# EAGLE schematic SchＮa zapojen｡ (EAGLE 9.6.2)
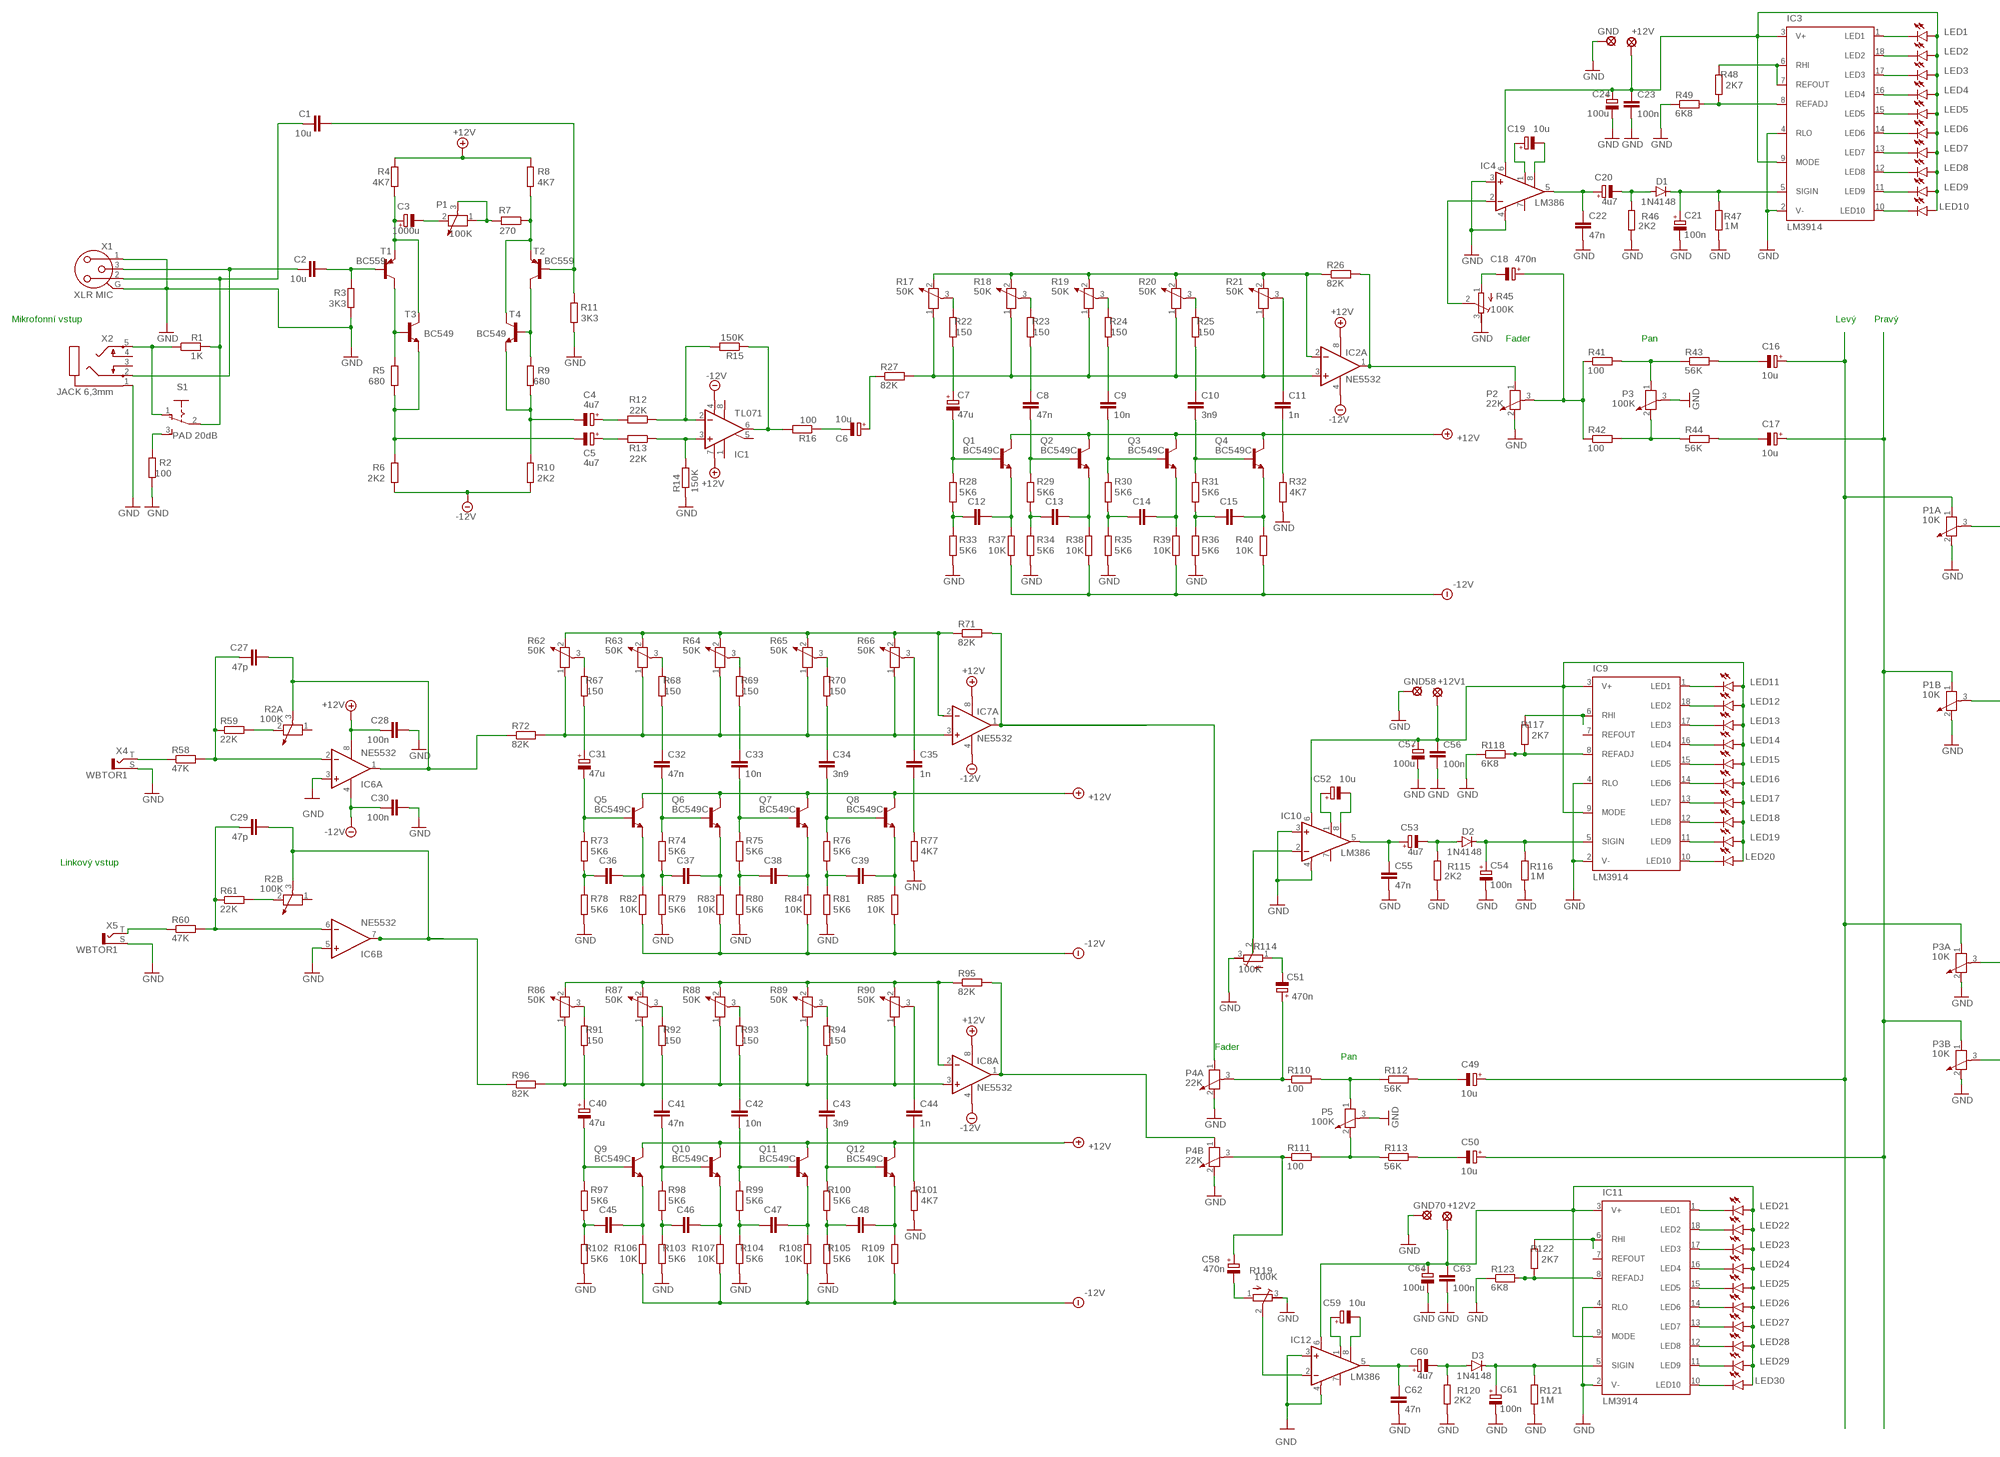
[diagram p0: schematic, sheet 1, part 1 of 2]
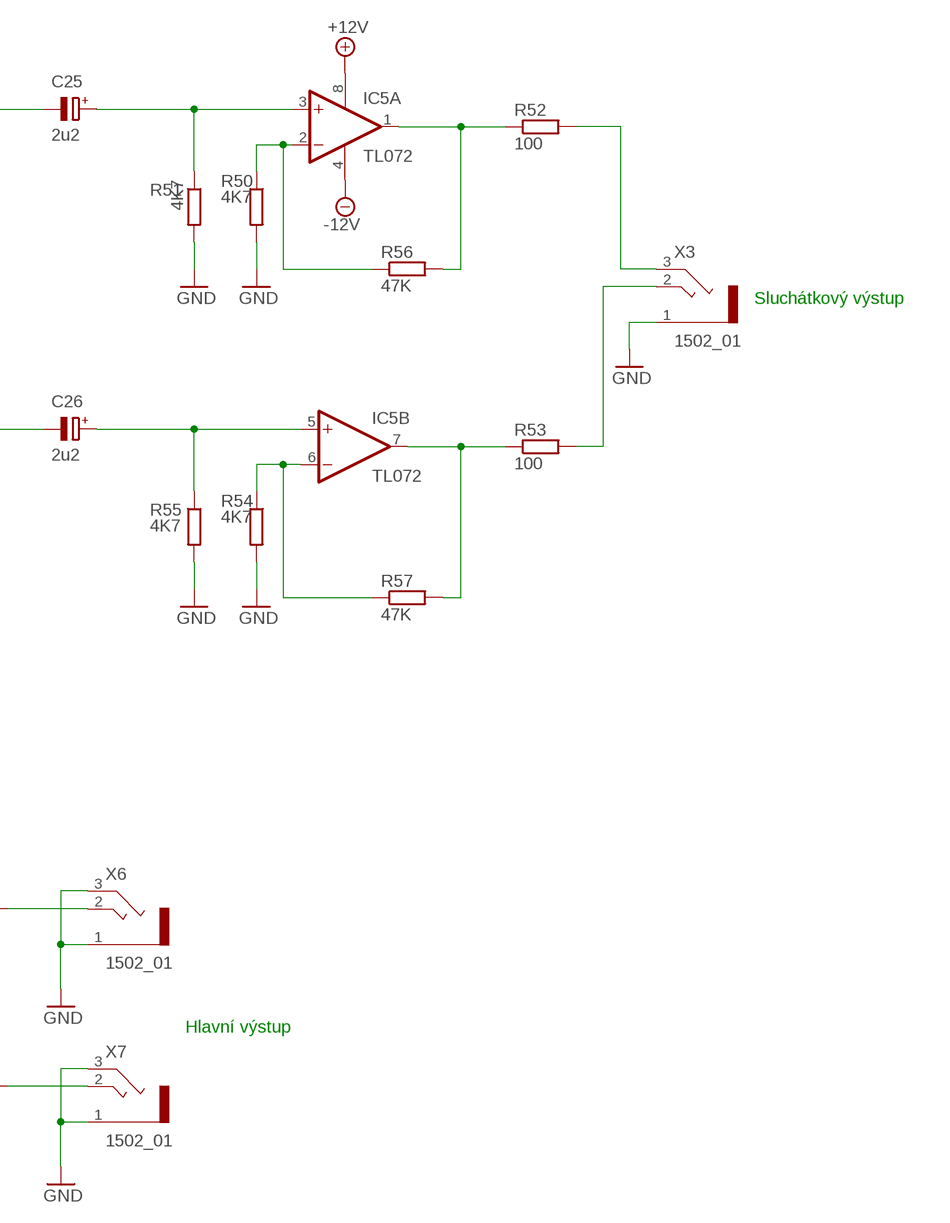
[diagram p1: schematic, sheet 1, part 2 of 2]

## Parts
+12V  MCS08  [MCS08]
+12V1  MCS08  [MCS08]
+12V2  MCS08  [MCS08]
C1  10u  C-EU050-025X075  [C050-025X075]
C2  10u  C-EU050-025X075  [C050-025X075]
C3  1000u  CPOL-EUE3.5-8  [E3,5-8]
C4  4u7  CPOL-EUE3.5-8  [E3,5-8]
C5  4u7  CPOL-EUE3.5-8  [E3,5-8]
C6  10u  CPOL-EUE3.5-8  [E3,5-8]
C7  47u  CPOL-EUE1.8-4  [E1,8-4]
C8  47n  C-EU050-030X075  [C050-030X075]
C9  10n  C-EU050-030X075  [C050-030X075]
C10  3n9  C-EU050-030X075  [C050-030X075]
C11  1n  C-EU050-030X075  [C050-030X075]
C12  C-EU050-030X075  [C050-030X075]
C13  C-EU050-030X075  [C050-030X075]
C14  C-EU050-030X075  [C050-030X075]
C15  C-EU050-030X075  [C050-030X075]
C16  10u  CPOL-EUE2.5-5  [E2,5-5]
C17  10u  CPOL-EUE2.5-5  [E2,5-5]
C18  470n  CPOL-EUE2.5-5  [E2,5-5]
C19  10u  CPOL-EUE2.5-5  [E2,5-5]
C20  4u7  CPOL-EUE2.5-5  [E2,5-5]
C21  100n  CPOL-EUE2.5-5  [E2,5-5]
C22  47n  C-EU050-030X075  [C050-030X075]
C23  100n  C-EU050-030X075  [C050-030X075]
C24  100u  CPOL-EUE2.5-5  [E2,5-5]
C25  2u2  CPOL-EUE2,5-6E  [E2,5-6E]
C26  2u2  CPOL-EUE2,5-6E  [E2,5-6E]
C27  47p  C-EU050-024X044  [C050-024X044]
C28  100n  C-EU050-024X044  [C050-024X044]
C29  47p  C-EU050-024X044  [C050-024X044]
C30  100n  C-EU050-024X044  [C050-024X044]
C31  47u  CPOL-EUE1.8-4  [E1,8-4]
C32  47n  C-EU050-030X075  [C050-030X075]
C33  10n  C-EU050-030X075  [C050-030X075]
C34  3n9  C-EU050-030X075  [C050-030X075]
C35  1n  C-EU050-030X075  [C050-030X075]
C36  C-EU050-030X075  [C050-030X075]
C37  C-EU050-030X075  [C050-030X075]
C38  C-EU050-030X075  [C050-030X075]
C39  C-EU050-030X075  [C050-030X075]
C40  47u  CPOL-EUE1.8-4  [E1,8-4]
C41  47n  C-EU050-030X075  [C050-030X075]
C42  10n  C-EU050-030X075  [C050-030X075]
C43  3n9  C-EU050-030X075  [C050-030X075]
C44  1n  C-EU050-030X075  [C050-030X075]
C45  C-EU050-030X075  [C050-030X075]
C46  C-EU050-030X075  [C050-030X075]
C47  C-EU050-030X075  [C050-030X075]
C48  C-EU050-030X075  [C050-030X075]
C49  10u  CPOL-EUE2.5-5  [E2,5-5]
C50  10u  CPOL-EUE2.5-5  [E2,5-5]
C51  470n  CPOL-EUE2.5-5  [E2,5-5]
C52  10u  CPOL-EUE2.5-5  [E2,5-5]
C53  4u7  CPOL-EUE2.5-5  [E2,5-5]
C54  100n  CPOL-EUE2.5-5  [E2,5-5]
C55  47n  C-EU050-030X075  [C050-030X075]
C56  100n  C-EU050-030X075  [C050-030X075]
C57  100u  CPOL-EUE2.5-5  [E2,5-5]
C58  470n  CPOL-EUE2.5-5  [E2,5-5]
C59  10u  CPOL-EUE2.5-5  [E2,5-5]
C60  4u7  CPOL-EUE2.5-5  [E2,5-5]
C61  100n  CPOL-EUE2.5-5  [E2,5-5]
C62  47n  C-EU050-030X075  [C050-030X075]
C63  100n  C-EU050-030X075  [C050-030X075]
C64  100u  CPOL-EUE2.5-5  [E2,5-5]
D1  1N4148  1N4148DO35-7  [DO35-7]
D2  1N4148  1N4148DO35-7  [DO35-7]
D3  1N4148  1N4148DO35-7  [DO35-7]
GND  MCS08  [MCS08]
GND58  MCS08  [MCS08]
GND70  MCS08  [MCS08]
IC1  TL071  TL071P  [DIL08]
IC2  NE5532  NE5532N  [DIL08]
IC3  LM3914  LM3914N  [DIL18]
IC4  LM386  LM386N-1  [DIL08]
IC5  TL072  TL072P  [DIL08]
IC6  NE5532  NE5532N  [DIL08]
IC7  NE5532  NE5532N  [DIL08]
IC8  NE5532  NE5532N  [DIL08]
IC9  LM3914  LM3914N  [DIL18]
IC10  LM386  LM386N-1  [DIL08]
IC11  LM3914  LM3914N  [DIL18]
IC12  LM386  LM386N-1  [DIL08]
LED1  LED10MM  [LED10MM]
LED2  LED10MM  [LED10MM]
LED3  LED10MM  [LED10MM]
LED4  LED10MM  [LED10MM]
LED5  LED10MM  [LED10MM]
LED6  LED10MM  [LED10MM]
LED7  LED10MM  [LED10MM]
LED8  LED10MM  [LED10MM]
LED9  LED10MM  [LED10MM]
LED10  LED10MM  [LED10MM]
LED11  LED10MM  [LED10MM]
LED12  LED10MM  [LED10MM]
LED13  LED10MM  [LED10MM]
LED14  LED10MM  [LED10MM]
LED15  LED10MM  [LED10MM]
LED16  LED10MM  [LED10MM]
LED17  LED10MM  [LED10MM]
LED18  LED10MM  [LED10MM]
LED19  LED10MM  [LED10MM]
LED20  LED10MM  [LED10MM]
LED21  LED10MM  [LED10MM]
LED22  LED10MM  [LED10MM]
LED23  LED10MM  [LED10MM]
LED24  LED10MM  [LED10MM]
LED25  LED10MM  [LED10MM]
LED26  LED10MM  [LED10MM]
LED27  LED10MM  [LED10MM]
LED28  LED10MM  [LED10MM]
LED29  LED10MM  [LED10MM]
LED30  LED10MM  [LED10MM]
P1  100K  POTENTIOMETER_PT-10  [PT-10]
P1A  10K  POTENTIOMETER_PT-10  [PT-10]
P1B  10K  POTENTIOMETER_PT-10  [PT-10]
P2  22K  POTENTIOMETER_PT-10  [PT-10]
P3  100K  POTENTIOMETER_PT-10  [PT-10]
P3A  10K  POTENTIOMETER_PT-10  [PT-10]
P3B  10K  POTENTIOMETER_PT-10  [PT-10]
P4A  22K  POTENTIOMETER_PT-10  [PT-10]
P4B  22K  POTENTIOMETER_PT-10  [PT-10]
P5  100K  POTENTIOMETER_PT-10  [PT-10]
Q1  BC549C  [TO92-EBC]
Q2  BC549C  [TO92-EBC]
Q3  BC549C  [TO92-EBC]
Q4  BC549C  [TO92-EBC]
Q5  BC549C  [TO92-EBC]
Q6  BC549C  [TO92-EBC]
Q7  BC549C  [TO92-EBC]
Q8  BC549C  [TO92-EBC]
Q9  BC549C  [TO92-EBC]
Q10  BC549C  [TO92-EBC]
Q11  BC549C  [TO92-EBC]
Q12  BC549C  [TO92-EBC]
R1  1K  R-EU_0207/7  [0207/7]
R2  100  R-EU_0207/7  [0207/7]
R2A  100K  POTENTIOMETER_PT-10  [PT-10]
R2B  100K  POTENTIOMETER_PT-10  [PT-10]
R3  3K3  R-EU_0207/7  [0207/7]
R4  4K7  R-EU_0207/7  [0207/7]
R5  680  R-EU_0207/7  [0207/7]
R6  2K2  R-EU_0207/7  [0207/7]
R7  270  R-EU_0207/7  [0207/7]
R8  4K7  R-EU_0207/7  [0207/7]
R9  680  R-EU_0207/7  [0207/7]
R10  2K2  R-EU_0207/7  [0207/7]
R11  3K3  R-EU_0207/7  [0207/7]
R12  22K  R-EU_0207/7  [0207/7]
R13  22K  R-EU_0207/7  [0207/7]
R14  150K  R-EU_0207/7  [0207/7]
R15  150K  R-EU_0207/7  [0207/7]
R16  100  R-EU_0207/7  [0207/7]
R17  50K  POTENTIOMETER_PT-10S  [PT-10S]
R18  50K  POTENTIOMETER_PT-10S  [PT-10S]
R19  50K  POTENTIOMETER_PT-10S  [PT-10S]
R20  50K  POTENTIOMETER_PT-10S  [PT-10S]
R21  50K  POTENTIOMETER_PT-10S  [PT-10S]
R22  150  R-EU_0207/7  [0207/7]
R23  150  R-EU_0207/7  [0207/7]
R24  150  R-EU_0207/7  [0207/7]
R25  150  R-EU_0207/7  [0207/7]
R26  82K  R-EU_0207/7  [0207/7]
R27  82K  R-EU_0207/7  [0207/7]
R28  5K6  R-EU_0207/7  [0207/7]
R29  5K6  R-EU_0207/7  [0207/7]
R30  5K6  R-EU_0207/7  [0207/7]
R31  5K6  R-EU_0207/7  [0207/7]
R32  4K7  R-EU_0207/7  [0207/7]
R33  5K6  R-EU_0207/7  [0207/7]
R34  5K6  R-EU_0207/7  [0207/7]
R35  5K6  R-EU_0207/7  [0207/7]
R36  5K6  R-EU_0207/7  [0207/7]
R37  10K  R-EU_0207/7  [0207/7]
R38  10K  R-EU_0207/7  [0207/7]
R39  10K  R-EU_0207/7  [0207/7]
R40  10K  R-EU_0207/7  [0207/7]
R41  100  R-EU_0207/10  [0207/10]
R42  100  R-EU_0207/10  [0207/10]
R43  56K  R-EU_0207/10  [0207/10]
R44  56K  R-EU_0207/10  [0207/10]
R45  100K  R-TRIMM74W  [RTRIM74W]
R46  2K2  R-EU_0204/7  [0204/7]
R47  1M  R-EU_0204/7  [0204/7]
R48  2K7  R-EU_0204/7  [0204/7]
R49  6K8  R-EU_0204/7  [0204/7]
R50  4K7  R-EU_0207/7  [0207/7]
R51  4K7  R-EU_0207/7  [0207/7]
R52  100  R-EU_0207/7  [0207/7]
R53  100  R-EU_0207/7  [0207/7]
R54  4K7  R-EU_0207/7  [0207/7]
R55  4K7  R-EU_0207/7  [0207/7]
R56  47K  R-EU_0207/7  [0207/7]
R57  47K  R-EU_0207/7  [0207/7]
R58  47K  R-EU_0207/7  [0207/7]
R59  22K  R-EU_0207/7  [0207/7]
R60  47K  R-EU_0207/7  [0207/7]
R61  22K  R-EU_0207/7  [0207/7]
R62  50K  POTENTIOMETER_PT-10S  [PT-10S]
R63  50K  POTENTIOMETER_PT-10S  [PT-10S]
R64  50K  POTENTIOMETER_PT-10S  [PT-10S]
R65  50K  POTENTIOMETER_PT-10S  [PT-10S]
R66  50K  POTENTIOMETER_PT-10S  [PT-10S]
R67  150  R-EU_0207/7  [0207/7]
R68  150  R-EU_0207/7  [0207/7]
R69  150  R-EU_0207/7  [0207/7]
R70  150  R-EU_0207/7  [0207/7]
R71  82K  R-EU_0207/7  [0207/7]
R72  82K  R-EU_0207/7  [0207/7]
R73  5K6  R-EU_0207/7  [0207/7]
R74  5K6  R-EU_0207/7  [0207/7]
R75  5K6  R-EU_0207/7  [0207/7]
R76  5K6  R-EU_0207/7  [0207/7]
R77  4K7  R-EU_0207/7  [0207/7]
R78  5K6  R-EU_0207/7  [0207/7]
R79  5K6  R-EU_0207/7  [0207/7]
R80  5K6  R-EU_0207/7  [0207/7]
R81  5K6  R-EU_0207/7  [0207/7]
R82  10K  R-EU_0207/7  [0207/7]
R83  10K  R-EU_0207/7  [0207/7]
R84  10K  R-EU_0207/7  [0207/7]
R85  10K  R-EU_0207/7  [0207/7]
R86  50K  POTENTIOMETER_PT-10S  [PT-10S]
R87  50K  POTENTIOMETER_PT-10S  [PT-10S]
R88  50K  POTENTIOMETER_PT-10S  [PT-10S]
R89  50K  POTENTIOMETER_PT-10S  [PT-10S]
R90  50K  POTENTIOMETER_PT-10S  [PT-10S]
R91  150  R-EU_0207/7  [0207/7]
R92  150  R-EU_0207/7  [0207/7]
R93  150  R-EU_0207/7  [0207/7]
R94  150  R-EU_0207/7  [0207/7]
R95  82K  R-EU_0207/7  [0207/7]
R96  82K  R-EU_0207/7  [0207/7]
R97  5K6  R-EU_0207/7  [0207/7]
R98  5K6  R-EU_0207/7  [0207/7]
R99  5K6  R-EU_0207/7  [0207/7]
R100  5K6  R-EU_0207/7  [0207/7]
R101  4K7  R-EU_0207/7  [0207/7]
R102  5K6  R-EU_0207/7  [0207/7]
R103  5K6  R-EU_0207/7  [0207/7]
R104  5K6  R-EU_0207/7  [0207/7]
R105  5K6  R-EU_0207/7  [0207/7]
R106  10K  R-EU_0207/7  [0207/7]
R107  10K  R-EU_0207/7  [0207/7]
R108  10K  R-EU_0207/7  [0207/7]
R109  10K  R-EU_0207/7  [0207/7]
R110  100  R-EU_0207/10  [0207/10]
R111  100  R-EU_0207/10  [0207/10]
R112  56K  R-EU_0207/10  [0207/10]
R113  56K  R-EU_0207/10  [0207/10]
R114  100K  R-TRIMM74W  [RTRIM74W]
R115  2K2  R-EU_0204/7  [0204/7]
R116  1M  R-EU_0204/7  [0204/7]
R117  2K7  R-EU_0204/7  [0204/7]
R118  6K8  R-EU_0204/7  [0204/7]
R119  100K  R-TRIMM74W  [RTRIM74W]
R120  2K2  R-EU_0204/7  [0204/7]
R121  1M  R-EU_0204/7  [0204/7]
R122  2K7  R-EU_0204/7  [0204/7]
R123  6K8  R-EU_0204/7  [0204/7]
S1  PAD 20dB  255SB  [255SB]
T1  BC559  BC559A-PNP-TO92-EBC  [TO92-EBC]
T2  BC559  BC559A-PNP-TO92-EBC  [TO92-EBC]
T3  BC549  BC549-NPN-TO92-CBE  [TO92-CBE]
T4  BC549  BC549-NPN-TO92-CBE  [TO92-CBE]
X1  XLR MIC  NC3FAV2  [NC3FAV2]
X2  JACK 6,3mm  PG203J  [PG203J]
X3  1502_01  [1502_01]
X4  WBTOR1  [WBTOR1]
X5  WBTOR1  [WBTOR1]
X6  1502_01  [1502_01]
X7  1502_01  [1502_01]

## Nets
+12V: C28.1 IC1.7(V+) IC2.8(P:V+) IC5.8(P:V+) IC6.8(P:V+) IC7.8(P:V+) IC8.8(P:V+) R4.2 R8.2
-12V: C30.1 IC1.4(V-) IC2.4(P:V-) IC5.4(P:V-) IC6.4(P:V-) IC7.4(P:V-) IC8.4(P:V-) R6.1 R10.1
GND: C21.- C22.2 C23.2 C24.- C28.2 C30.2 C54.- C55.2 C61.- C62.2 GND.MP IC3.2(V-) IC3.4(RLO) IC4.3(+IN) IC4.4(GND) IC6.3(A:+IN) IC6.5(B:+IN) P1A.2 P1B.2 P2.2 P3.3 P3A.2 P3B.2 P4A.2 P4B.2 P5.3 R2.1 R3.1 R11.1 R14.1 R32.1 R33.1 R34.1 R35.1 R36.1 R45.3(E) R46.1 R47.1 R49.1 R50.2 R51.2 R54.2 R55.2 R77.1 R78.1 R79.1 R80.1 R81.1 R101.1 R102.1 R103.1 R104.1 R105.1 R114.3(E) R115.1 R116.1 R119.3(E) R120.1 R121.1 X1.1 X1.G X2.1 X3.1 X4.S X5.S X6.1 X6.3 X7.1 X7.3
GND1: C56.2 C57.- GND58.MP IC9.2(V-) IC9.4(RLO) IC10.3(+IN) IC10.4(GND) R118.1 ; supply symbol labelled GND
GND2: C63.2 C64.- GND70.MP IC11.2(V-) IC11.4(RLO) IC12.3(+IN) IC12.4(GND) R123.1 ; supply symbol labelled GND
N$1: C6.+ R27.1
N$2: R2.2 S1.3(S)
N$3: C2.1 X1.3 X2.2
N$4: C1.1 R1.2 S1.2(P) X1.2
N$5: R1.1 S1.1(O) X2.5
N$6: R17.3 R22.2
N$7: C2.2 R3.2 T1.B
N$8: R5.2 T1.C T3.B
N$9: R9.2 T2.C T4.B
N$10: C1.2 R11.2 T2.B
N$11: R18.3 R23.2
N$12: R7.1 R8.1 T2.E T4.C
N$13: C3.+ R4.1 T1.E T3.C
N$14: C5.- R5.1 R6.2 T3.E
N$15: R19.3 R24.2
N$16: C4.- R9.1 R10.2 T4.E
N$17: C3.- P1.2
N$18: P1.1 P1.3 R7.2
N$19: C4.+ R12.2
N$20: C5.+ R13.2
N$21: IC1.2(-IN) R12.1 R15.2
N$22: IC1.3(+IN) R13.1 R14.2
N$23: C6.- R16.1
N$24: IC1.6(OUT) R15.1 R16.2
N$25: R20.3 R25.2
N$26: C7.+ R22.1
N$27: R17.1 R18.1 R19.1 R20.1 R21.1 R27.2
N$28: C8.1 R23.1
N$29: C9.1 R24.1
N$30: C10.1 R25.1
N$31: C7.- Q1.B R28.2
N$32: C8.2 Q2.B R29.2
N$33: C9.2 Q3.B R30.2
N$34: C10.2 Q4.B R31.2
N$35: C15.2 Q4.E R40.2
N$36: C14.2 Q3.E R39.2
N$37: C13.2 Q2.E R38.2
N$38: C12.2 Q1.E R37.2
N$39: C12.1 R28.1 R33.2
N$40: C13.1 R29.1 R34.2
N$41: C14.1 R30.1 R35.2
N$42: C15.1 R31.1 R36.2
N$43: C11.2 R32.2
N$44: R17.2 R18.2 R19.2 R20.2 R21.2 R26.1
N$45: Q1.C Q2.C Q3.C Q4.C
N$46: R37.1 R38.1 R39.1 R40.1
N$47: C51.+ P4A.3 R110.1
N$48: IC2.1(A:OUT) P2.1 R26.2
N$49: C11.1 R21.3
N$50: P3A.3 X6.2
N$51: P3.1 R41.2 R43.1
N$52: P3.2 R42.2 R44.1
N$53: C16.- R43.2
N$54: C17.- R44.2
N$55: P3B.3 X7.2
N$56: R62.3 R67.2
N$57: C58.+ P4B.3 R111.1
N$58: C19.+ IC4.1(GAIN)
N$59: C19.- IC4.8(GAIN)
N$60: C20.+ C22.1 IC4.5(OUT)
N$61: C20.- D1.A R46.2
N$62: C21.+ D1.C IC3.5(SIGIN) R47.2
N$63: IC4.2(-IN) R45.2(S)
N$64: C18.- R45.1(A)
N$65: C18.+ P2.3 R41.1 R42.1
N$66: IC3.8(REFADJ) R48.1 R49.2
N$67: IC3.6(RHI) IC3.7(REFOUT) R48.2
N$68: +12V.MP C23.1 C24.+ IC3.3(V+) IC3.9(MODE) IC4.6(VS) LED1.A LED2.A LED3.A LED4.A LED5.A LED6.A LED7.A LED8.A LED9.A LED10.A
N$69: IC3.1(LED1) LED1.K(C)
N$70: IC3.18(LED2) LED2.K(C)
N$71: IC3.17(LED3) LED3.K(C)
N$72: IC3.16(LED4) LED4.K(C)
N$73: IC3.15(LED5) LED5.K(C)
N$74: IC3.14(LED6) LED6.K(C)
N$75: IC3.13(LED7) LED7.K(C)
N$76: IC3.12(LED8) LED8.K(C)
N$77: IC3.11(LED9) LED9.K(C)
N$78: IC3.10(LED10) LED10.K(C)
N$79: C26.- P1B.3
N$80: C25.- P1A.3
N$81: C25.+ IC5.3(A:+IN) R51.1
N$82: C26.+ IC5.5(B:+IN) R55.1
N$83: IC5.2(A:-IN) R50.1 R56.1
N$84: IC5.1(A:OUT) R52.1 R56.2
N$85: IC5.7(B:OUT) R53.1 R57.2
N$86: IC5.6(B:-IN) R54.1 R57.1
N$87: R53.2 X3.2
N$88: R52.2 X3.3
N$89: R63.3 R68.2
N$90: R64.3 R69.2
N$91: C27.1 IC6.2(A:-IN) R58.2 R59.1
N$92: C29.1 IC6.6(B:-IN) R60.2 R61.1
N$93: R2A.2 R59.2
N$94: R2B.2 R61.2
N$95: C27.2 IC6.1(A:OUT) R2A.3 R72.1
N$96: C29.2 IC6.7(B:OUT) R2B.3 R96.1
N$97: R58.1 X4.T
N$98: R60.1 X5.T
N$99: R65.3 R70.2
N$100: C31.+ R67.1
N$101: R62.1 R63.1 R64.1 R65.1 R66.1 R72.2
N$102: C32.1 R68.1
N$103: C33.1 R69.1
N$104: C34.1 R70.1
N$105: C31.- Q5.B R73.2
N$106: C32.2 Q6.B R74.2
N$107: C33.2 Q7.B R75.2
N$108: C34.2 Q8.B R76.2
N$109: C39.2 Q8.E R85.2
N$110: C38.2 Q7.E R84.2
N$111: C37.2 Q6.E R83.2
N$112: C36.2 Q5.E R82.2
N$113: C36.1 R73.1 R78.2
N$114: C37.1 R74.1 R79.2
N$115: C38.1 R75.1 R80.2
N$116: C39.1 R76.1 R81.2
N$117: C35.2 R77.2
N$118: R62.2 R63.2 R64.2 R65.2 R66.2 R71.1
N$119: Q5.C Q6.C Q7.C Q8.C
N$120: R82.1 R83.1 R84.1 R85.1
N$121: IC7.1(A:OUT) P4A.1 R71.2
N$122: C35.1 R66.3
N$123: C59.+ IC12.1(GAIN)
N$124: R86.3 R91.2
N$125: R87.3 R92.2
N$126: R88.3 R93.2
N$127: R89.3 R94.2
N$128: C40.+ R91.1
N$129: R86.1 R87.1 R88.1 R89.1 R90.1 R96.2
N$130: C41.1 R92.1
N$131: C42.1 R93.1
N$132: C43.1 R94.1
N$133: C40.- Q9.B R97.2
N$134: C41.2 Q10.B R98.2
N$135: C42.2 Q11.B R99.2
N$136: C43.2 Q12.B R100.2
N$137: C48.2 Q12.E R109.2
N$138: C47.2 Q11.E R108.2
N$139: C46.2 Q10.E R107.2
N$140: C45.2 Q9.E R106.2
N$141: C45.1 R97.1 R102.2
N$142: C46.1 R98.1 R103.2
N$143: C47.1 R99.1 R104.2
N$144: C48.1 R100.1 R105.2
N$145: C44.2 R101.2
N$146: R86.2 R87.2 R88.2 R89.2 R90.2 R95.1
N$147: Q9.C Q10.C Q11.C Q12.C
N$148: R106.1 R107.1 R108.1 R109.1
N$149: IC8.1(A:OUT) P4B.1 R95.2
N$150: C44.1 R90.3
N$151: P5.1 R110.2 R112.1
N$152: P5.2 R111.2 R113.1
N$153: C49.- R112.2
N$154: C50.- R113.2
N$156: C17.+ C50.+ P1B.1 P3B.1
N$157: C16.+ C49.+ P1A.1 P3A.1
N$158: C52.+ IC10.1(GAIN)
N$159: C52.- IC10.8(GAIN)
N$160: C53.+ C55.1 IC10.5(OUT)
N$161: C53.- D2.A R115.2
N$162: C54.+ D2.C IC9.5(SIGIN) R116.2
N$163: IC10.2(-IN) R114.2(S)
N$164: C51.- R114.1(A)
N$166: IC9.8(REFADJ) R117.1 R118.2
N$167: IC9.6(RHI) R117.2
N$168: +12V1.MP C56.1 C57.+ IC9.3(V+) IC9.9(MODE) IC10.6(VS) LED11.A LED12.A LED13.A LED14.A LED15.A LED16.A LED17.A LED18.A LED19.A LED20.A
N$169: IC9.1(LED1) LED11.K(C)
N$170: IC9.18(LED2) LED12.K(C)
N$171: IC9.17(LED3) LED13.K(C)
N$172: IC9.16(LED4) LED14.K(C)
N$173: IC9.15(LED5) LED15.K(C)
N$174: IC9.14(LED6) LED16.K(C)
N$175: IC9.13(LED7) LED17.K(C)
N$176: IC9.12(LED8) LED18.K(C)
N$177: IC9.11(LED9) LED19.K(C)
N$178: IC9.10(LED10) LED20.K(C)
N$180: C59.- IC12.8(GAIN)
N$181: C60.+ C62.1 IC12.5(OUT)
N$182: C60.- D3.A R120.2
N$183: C61.+ D3.C IC11.5(SIGIN) R121.2
N$184: IC12.2(-IN) R119.2(S)
N$185: C58.- R119.1(A)
N$187: IC11.8(REFADJ) R122.1 R123.2
N$188: IC11.6(RHI) R122.2
N$189: +12V2.MP C63.1 C64.+ IC11.3(V+) IC11.9(MODE) IC12.6(VS) LED21.A LED22.A LED23.A LED24.A LED25.A LED26.A LED27.A LED28.A LED29.A LED30.A
N$190: IC11.1(LED1) LED21.K(C)
N$191: IC11.18(LED2) LED22.K(C)
N$192: IC11.17(LED3) LED23.K(C)
N$193: IC11.16(LED4) LED24.K(C)
N$194: IC11.15(LED5) LED25.K(C)
N$195: IC11.14(LED6) LED26.K(C)
N$196: IC11.13(LED7) LED27.K(C)
N$197: IC11.12(LED8) LED28.K(C)
N$198: IC11.11(LED9) LED29.K(C)
N$199: IC11.10(LED10) LED30.K(C)
Unconnected: IC1.1(ON1) IC1.5(ON2) IC1.8(OPT) IC2.2(A:-IN) IC2.3(A:+IN) IC2.5(B:+IN) IC2.6(B:-IN) IC2.7(B:OUT) IC4.7(BYPASS) IC7.2(A:-IN) IC7.3(A:+IN) IC7.5(B:+IN) IC7.6(B:-IN) IC7.7(B:OUT) IC8.2(A:-IN) IC8.3(A:+IN) IC8.5(B:+IN) IC8.6(B:-IN) IC8.7(B:OUT) IC9.7(REFOUT) IC10.7(BYPASS) IC11.7(REFOUT) IC12.7(BYPASS) R2A.1 R2B.1 X2.3 X2.4

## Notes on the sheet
- Mikrofonní vstup | Levý | Pravý
- Fader | Pan
- Sluchátkový výstup
- Linkový vstup
- Hlavní výstup
- Fader
- Pan

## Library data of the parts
+12V +12V1 +12V2 GND GND58 GND70 = solpad:MCS08: SOLDER PAD
C1 C2 C8-C15 C22 C23 C27-C30 C32-C39 C41-C48 C55 C56 C62 C63 = rcl:C-EU: CAPACITOR, European symbol; SPICEPREFIX: C
C3-C7 C16-C21 C24-C26 C31 C40 C49-C54 C57-C61 C64 = rcl:CPOL-EU: POLARIZED CAPACITOR, European symbol; SPICEPREFIX: C
D1-D3 = diode:1N4148: DIODE
IC1 = linear:TL071: OP AMP
IC2 IC6-IC8 = linear:NE5532: AUDIO AMPLIFIER
IC3 IC9 IC11 = national-semiconductor:LM391: Dot/Bar Display Driver Source: Data sheet LM3915 Data sheet LM3914
IC4 IC10 IC12 = linear:LM386?-*: Low Voltage Audio Power Amplifier Source: http://cache.national.com/ds/LM/LM386.pdf
IC5 = linear:TL072: OP AMP
LED1-LED30 = led:LED: LED
P1 P1A P1B P2 P3 P3A P3B P4A P4B P5 R2A R2B R17-R21 R62-R66 R86-R90 = rcl:POTENTIOMETER_: Potentiometer; SPICEMODEL: POT; SPICEPREFIX: X
Q1-Q12 = transistor-npn:BC549*: NPN Transistor
R1-R16 R22-R44 R46-R61 R67-R85 R91-R113 R115-R118 R120-R123 = rcl:R-EU_: RESISTOR, European symbol; SPICEPREFIX: R
R45 R114 R119 = rcl:R-TRIMM: Trimm resistor; SPICEMODEL: X; SPICEPREFIXL: POT
S1 = switch:255SB: SLIDING SWITCH Distributor Buerklin, 11G810
T1 T2 = transistor:*-PNP-: PNP Transistror
T3 T4 = transistor:*-NPN-: NPN Transistror BF959 corrected 2008.03.06
X1 = con-neutrik_ag:NC3: Neutrik Audio Connector XLR SERIES Stereo 1/4" jack Source: www.neutrik.com/; MF: NEUTRIK; MPN: NC3FAV2; OC_FARNELL: unknown; OC_NEWARK: 83F7211
X2 = con-hirschmann:PG203J: MIC/HEADPHONE JACK KS-S stereo microphone/headphone jack PG203JN (Schukat); OC_FARNELL: unknown; OC_NEWARK: unknown
X3 X6 X7 = con-lumberg:1502_01: Jack connectors according to JISC 6560, 3.5 mm Klinkensteckverbinder nach JISC 6560, 3,5 mm Source: http://www.lumberg.com/Produkte/PDFs/1502_01.pdf; OC_FARNELL: 4739747; OC_NEWARK: unknown
X4 X5 = con-lumberg:WBTOR1: RCA connectors according to JEITA RC-5231 Cinch; MPN: WBTOR 1 BLACK; OC_FARNELL: 1200146; OC_NEWARK: 98K2588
